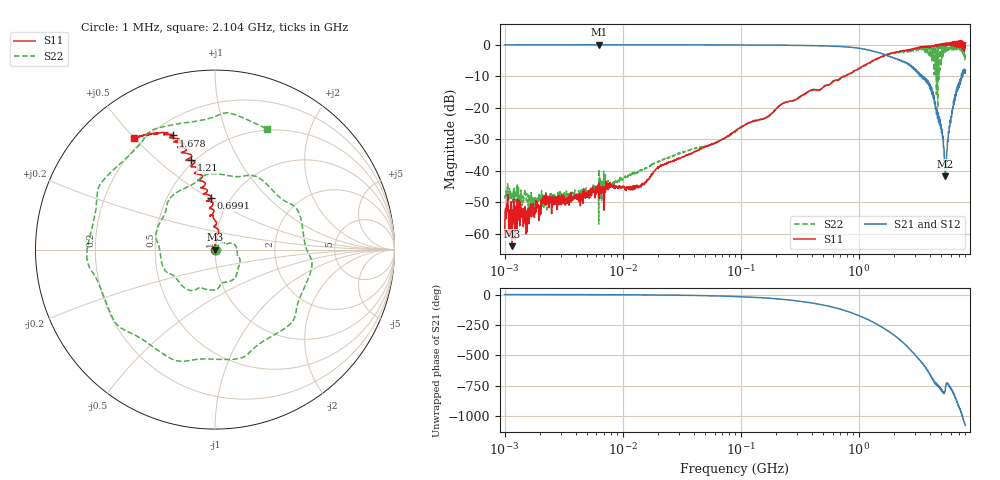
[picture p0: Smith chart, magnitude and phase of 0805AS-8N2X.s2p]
!s-Parameter Generated by FASTRON Sdn. Bhd.
!FASTRON P/N : 0805AS-8N2X
!Keysight Technologies: E5071C_MY46733604_B.14.02
!Date: Mon Jun 15 12:48:19 2026
!Version  :Rev01  Mon Jun 15 12:48:19 2026
!Data & Calibration Information:
!Freq  S11:SOLT2(ON)  S21:SOLT2(ON)  S12:SOLT2(ON)  S22:SOLT2(ON)
!PortZ  Port1:50+j0  Port2:50+j0
!When reading reference impedance value at option line is always used.
! Remarks : This data is being provided solely for informational purposes.
# Hz S dB R 50
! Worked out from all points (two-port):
!   1601 points, 1 MHz to 8 GHz, reference 50 ohm
!   highest |S21| = 0.02 dB at 6.301 MHz (marker M1); lowest = -41.8 dB at 5.416 GHz (marker M2)
!   |S21| within 3 dB of the highest: start of sweep to 1.63 GHz
!   lowest |S11| = -63.9 dB at 1.152 MHz (marker M3), VSWR 1.00, Z = 50.1 + j0.0179 ohm
!   |S11| at or under -10 dB: start of sweep to 744 MHz
!   |S22| runs from -56.9 to -0.3 dB; largest |S21 - S12| = 0.016
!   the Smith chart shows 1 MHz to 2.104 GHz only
!   S11 on the Smith chart (normalised r, x): 1 MHz: 1.00, +0.00; 699.1 MHz: 0.81, +0.51; 1.21 GHz: 0.48, +0.65; 1.678 GHz: 0.28, +0.66; 2.104 GHz: 0.16, +0.50
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1000000  -60.80 25.7  -0.06 -0.2  -0.03 -0.2  -48.80 8.7
1151819  -63.90 16.3  -0.06 -0.3  -0.02 -0.2  -47.10 10.2
4479405  -49.00 39.2  -0.04 -0.8  -0.03 -0.9  -47.90 42.2
6301378  -43.90 46.0  0.02 -1.3  -0.03 -1.2  -39.50 44.2
2.00676e7  -38.90 76.0  -0.05 -3.6  -0.05 -3.5  -37.10 60.2
8.994653e7  -27.30 79.5  -0.07 -15.9  -0.08 -15.9  -27.60 51.3
4.006501e8  -14.40 93.4  -0.30 -69.4  -0.30 -69.4  -14.30 -54.6
6.991365e8  -10.80 94.5  -0.60 -121.0  -0.60 -121.0  -10.50 -156.0
1.210338e9  -5.77 105.0  -1.71 151.0  -1.72 151.0  -5.92 16.8
1.677723e9  -3.39 110.0  -3.35 74.1  -3.33 73.9  -3.24 -144.0
1.7949e9  -2.92 114.0  -3.67 56.0  -3.66 55.8  -3.04 176.0
2.103821e9  -2.28 126.0  -4.43 6.9  -4.43 6.7  -2.71 66.8
2.545586e9  -1.88 137.0  -6.04 -64.0  -6.05 -64.0  -1.77 -85.9
3.029771e9  -1.19 143.0  -8.42 -142.0  -8.42 -142.0  -1.10 108.0
3.304817e9  -0.70 154.0  -9.81 174.0  -9.82 174.0  -1.08 7.3
3.568312e9  -0.70 172.0  -10.20 135.0  -10.10 134.0  -2.25 -88.5
4.054764e9  -0.54 180.0  -13.00 51.3  -13.00 50.5  -4.12 96.6
4.716529e9  -0.25 -159.0  -23.10 -39.9  -23.20 -41.0  -1.10 -93.8
5.416325e9  0.05 -135.0  -41.80 -53.6  -41.80 -53.8  -0.49 32.7
6.033702e9  0.73 -96.4  -22.90 -50.4  -22.90 -50.2  -1.35 -164.0
7.421677e9  0.58 -42.5  -9.28 99.8  -9.36 100.0  -2.14 88.5
8e9  0.60 -38.6  -7.91 1.1  -7.69 1.8  -4.56 -105.0
